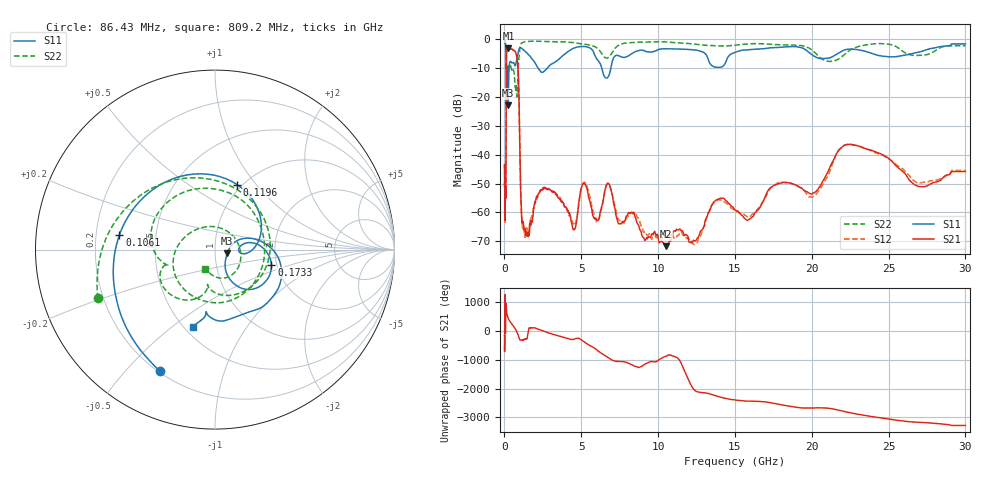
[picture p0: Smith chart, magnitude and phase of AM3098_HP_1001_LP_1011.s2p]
! Date/Time: Thu, Feb 28, 2019 8:41 AM
! Network Analyzer: Agilent Technologies E8364B Rev: A.07.50.67
! Sweep from 0.010 to 30.000 GHz, 1601 Points, Sweep Type: LOG
! Power Supply: 5.022 V, 0.002 A
# Hz S DB R 50
!freq MagS11 AngS11 MagS21 AngS21 MagS12 AngS12 MagS22 AngS22
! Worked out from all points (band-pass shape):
!   1601 points, 10 MHz to 30 GHz, reference 50 ohm
!   highest |S21| = -3.10 dB at 261.2 MHz (marker M1); lowest = -71.7 dB at 10.49 GHz (marker M2)
!   |S21| within 3 dB of the highest: 130.2 MHz to 805.6 MHz (675.4 MHz wide, 144 % of centre)
!   lowest |S11| = -22.9 dB at 239.9 MHz (marker M3), VSWR 1.15, Z = 57.3 - j2.33 ohm
!   |S11| at or under -10 dB: 191.7 MHz to 301.3 MHz (109.7 MHz wide, 44.5 % of centre); 2.194 GHz to 2.78 GHz (586.4 MHz wide, 23.6 % of centre); 6.337 GHz to 6.923 GHz (586 MHz wide, 8.84 % of centre)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
!   |S22| runs from -19.9 to -0.6 dB; largest |S21 - S12| = 0.012
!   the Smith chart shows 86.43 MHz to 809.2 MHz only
!   S11 on the Smith chart (normalised r, x): 86.43 MHz: 0.21, -0.63; 106.1 MHz: 0.30, +0.07; 119.6 MHz: 0.95, +0.80; 173.3 MHz: 1.87, -0.36; 809.2 MHz: 0.55, -0.59
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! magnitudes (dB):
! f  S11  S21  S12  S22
! 10 MHz  -0.3  -44.2  -47.8  -0.6
! 38.04 MHz  -0.5  -62.7  -61.4  -1.0
! 86.43 MHz  -2.6  -54.1  -52.7  -3.0
! 106.1 MHz  -5.4  -28.5  -28.5  -6.9
! 119.6 MHz  -8.3  -11.4  -11.4  -10.4
! 144.7 MHz  -17.2  -4.4  -4.4  -13.5
! 173.3 MHz  -9.7  -3.8  -3.8  -9.3
! 239.9 MHz  -22.9  -3.1  -3.1  -11.2
! 261.2 MHz  -16.4  -3.1  -3.0  -10.7
! 550.5 MHz  -8.0  -3.7  -3.6  -10.6
! 809.2 MHz  -7.0  -6.2  -6.2  -18.4
! 917.1 MHz  -4.0  -14.2  -14.2  -7.9
! 1.166 GHz  -3.3  -63.1  -64.7  -1.1
! 2.084 GHz  -9.0  -54.5  -55.8  -0.6
! 4.525 GHz  -3.0  -66.1  -64.4  -1.0
! 5.128 GHz  -2.4  -50.0  -49.7  -1.6
! 6.753 GHz  -13.0  -49.9  -50.0  -6.3
! 7.926 GHz  -6.1  -61.4  -63.0  -1.2
! 10.49 GHz  -3.2  -71.7  -68.2  -0.8
! 20.1 GHz  -5.6  -53.2  -54.4  -4.1
! 22.56 GHz  -3.4  -36.4  -36.4  -3.5
! 30 GHz  -1.6  -45.8  -45.4  -2.2
